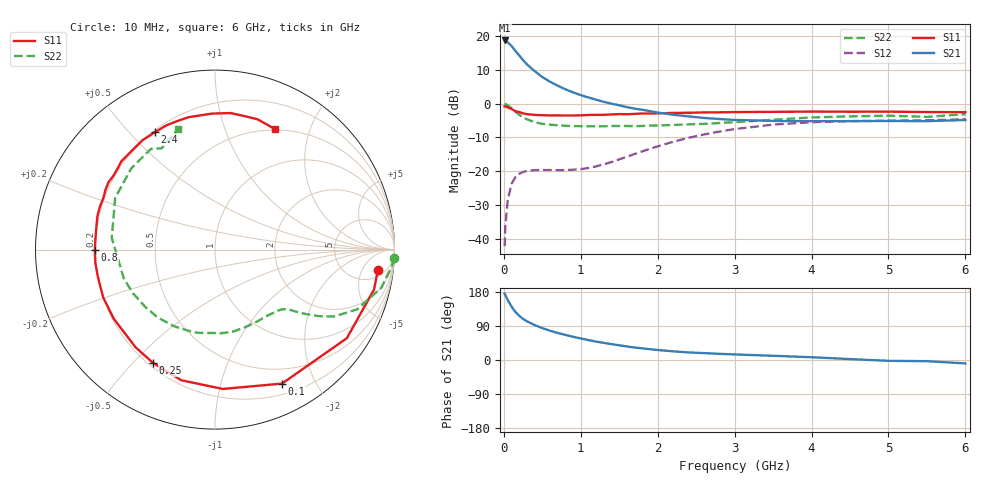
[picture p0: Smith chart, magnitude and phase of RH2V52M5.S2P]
! SIEMENS Small Signal Semiconductors
! BFR106
! Si NPN RF Bipolar Junction Transistor in SOT23
! VCE = 2.5 V  IC = 2.5 mA
! Common Emitter S-Parameters:  August  1996
# GHz  S  MA  R  50
!  f  S11  S21  S12  S22
! GHz  MAG  ANG  MAG  ANG  MAG  ANG  MAG  ANG
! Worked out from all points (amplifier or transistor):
!   36 points, 10 MHz to 6 GHz, reference 50 ohm
!   highest |S21| = 18.8 dB at 10 MHz (marker M1)
!   |S21| within 3 dB of that: start of sweep to 146.8 MHz
!   unconditionally stable (mu >= 1): 740.6 MHz to 2.087 GHz; 3.711 GHz to end of sweep
!   at 250 MHz: K = 0.36, MSG = 16.6 dB, |S12| = -20.3 dB
!   at 1.4 GHz: K = 1.25, MAG = 5.6 dB, |S12| = -17.3 dB
!   at 6 GHz: K = 1.02, MAG = -1.0 dB, |S12| = -4.6 dB
!   S11 on the Smith chart (normalised r, x): 10 MHz: 8, -11; 100 MHz: 0.32, -1.57; 250 MHz: 0.22, -0.57; 800 MHz: 0.20, -0.00; 2.4 GHz: 0.21, +0.59; 6 GHz: 0.49, +1.51
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0.01  0.915 -7.0  8.695 175.0  0.0077 87.2  0.9976 -2.8
0.02  0.9135 -14.1  8.634 171.3  0.0152 83.2  0.9896 -5.4
0.05  0.885 -33.9  8.201 158.2  0.0368 71.7  0.9508 -12.9
0.1  0.8347 -63.4  7.198 141.2  0.0646 57.5  0.8593 -22.8
0.15  0.7777 -86.8  6.091 126.6  0.0816 46.1  0.7612 -29.3
0.2  0.7517 -104.5  5.212 116.8  0.0914 39.3  0.6862 -32.7
0.25  0.7198 -118.6  4.442 108.2  0.0971 34.3  0.6258 -35.1
0.3  0.7016 -129.1  3.85 102.2  0.1009 31.3  0.5886 -36.7
0.4  0.6831 -145.7  3.053 92.3  0.1033 27.5  0.5331 -38.9
0.5  0.6774 -156.9  2.491 84.1  0.1037 26.7  0.5035 -41.2
0.6  0.6701 -166.3  2.122 77.3  0.1038 27.3  0.4888 -44.0
0.8  0.6696 -179.9  1.639 66.2  0.1036 32.2  0.4713 -50.8
1.1  0.6816 163.9  1.24 52.5  0.1114 44.7  0.4634 -63.1
1.6  0.6995 143.8  0.89 35.7  0.1636 60.9  0.4674 -86.6
2.2  0.7314 123.6  0.687 22.8  0.2724 60.3  0.4844 -118.3
2.4  0.7345 117.2  0.65 20.0  0.3121 57.4  0.4949 -130.1
3  0.7522 101.4  0.575 14.7  0.421 45.2  0.5329 -162.3
3.5  0.758 91.2  0.557 11.1  0.4903 33.9  0.579 173.5
4.5  0.7618 77.4  0.552 2.4  0.5516 13.7  0.6499 135.9
5  0.7636 71.9  0.555 -2.2  0.5617 6.0  0.6652 122.4
5.5  0.7533 66.7  0.552 -3.1  0.5673 2.4  0.6381 117.8
6  0.7498 63.3  0.573 -9.0  0.5898 -5.2  0.7012 107.2
